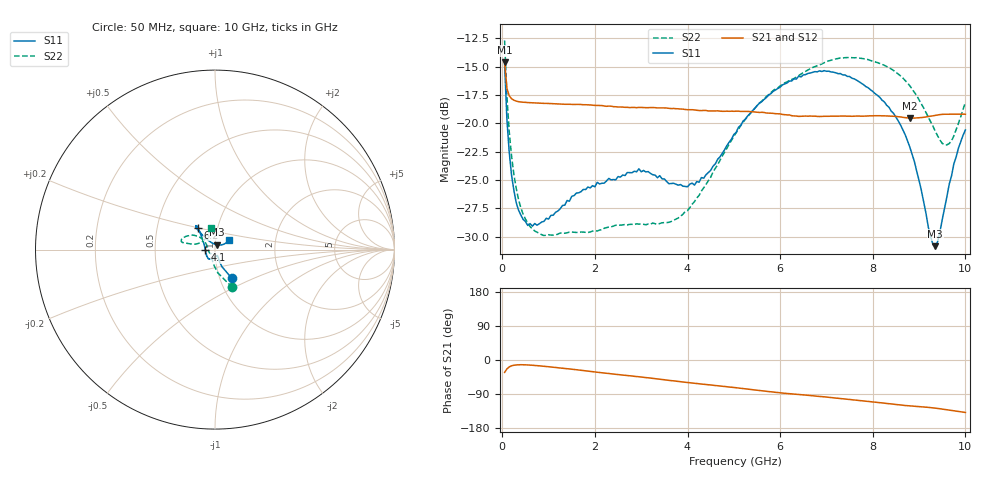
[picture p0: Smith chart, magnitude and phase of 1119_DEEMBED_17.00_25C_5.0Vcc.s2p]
!Hittite Microwave Corp.
!Digital Attenuator/PhaseShifter Rev 1.4.0
!Filename: C:\DATA\DATA\1119_DEEMBED_17.00_25C_5.0Vcc.s2p
!VNA ID: Agilent Technologies,N5224A,MY51441122,A.10.45.03
!Device type:
!2 Port Calibration.
!Temp(C): 25
!Lot Number:
!Serial Number:
!Operator:
!Misc:
!Attenuator:  17.000
# GHZ S DB R 50.0
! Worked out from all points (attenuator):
!   200 points, 50 MHz to 10 GHz, reference 50 ohm
!   highest |S21| = -14.61 dB at 50 MHz (marker M1); lowest = -19.5 dB at 8.8 GHz (marker M2)
!   lowest |S11| = -30.8 dB at 9.35 GHz (marker M3), VSWR 1.06, Z = 50.8 + j2.79 ohm
!   |S11| at or under -10 dB: start of sweep to end of sweep
!   |S22| runs from -29.9 to -12.7 dB; largest |S21 - S12| = 0.00046
!   S11 on the Smith chart (normalised r, x): 50 MHz: 1.14, -0.37; 4.1 GHz: 0.90, -0.00; 6.2 GHz: 0.81, +0.20; 10 GHz: 1.16, +0.12
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0.05  -14.75 -59.7  -14.61 -32.7  -14.61 -32.8  -12.68 -65.4
0.1  -19.67 -67.7  -16.91 -23.5  -16.91 -23.5  -17.62 -82.7
0.2  -24.57 -68.9  -17.82 -15.3  -17.82 -15.3  -22.90 -99.5
0.3  -26.98 -67.6  -18.03 -13.0  -18.02 -13.0  -25.71 -109.2
0.45  -28.47 -66.8  -18.13 -12.6  -18.13 -12.6  -28.01 -119.8
0.9  -28.64 -78.5  -18.23 -16.5  -18.25 -16.7  -29.89 -133.6
1.75  -25.82 -104.6  -18.35 -27.9  -18.35 -27.9  -29.59 -138.1
2.95  -24.00 -126.2  -18.59 -44.2  -18.60 -44.3  -28.89 -157.2
3.4  -24.61 -143.0  -18.63 -50.7  -18.63 -50.7  -28.83 -170.4
4.1  -25.27 -179.1  -18.79 -60.7  -18.80 -60.7  -27.13 161.4
4.5  -24.14 160.5  -18.90 -65.9  -18.92 -66.0  -24.75 147.4
5.05  -20.79 139.9  -18.92 -73.2  -18.94 -73.2  -20.82 140.5
5.55  -18.22 131.7  -19.03 -80.4  -19.04 -80.4  -18.21 142.6
6.2  -16.26 127.5  -19.25 -89.2  -19.27 -89.2  -16.20 148.4
6.7  -15.50 128.4  -19.36 -94.5  -19.37 -94.5  -15.07 154.9
7.5  -15.86 130.8  -19.36 -104.2  -19.37 -104.2  -14.19 163.9
8.35  -18.57 130.8  -19.35 -115.4  -19.35 -115.4  -15.08 167.5
8.8  -22.09 128.2  -19.53 -121.0  -19.52 -121.0  -16.68 167.2
9.25  -29.98 97.0  -19.36 -125.6  -19.38 -125.6  -19.86 160.9
9.35  -30.83 72.7  -19.29 -127.0  -19.31 -127.0  -20.69 155.8
9.65  -25.38 32.3  -19.19 -132.1  -19.20 -132.1  -21.78 126.5
10  -20.58 34.2  -19.19 -138.4  -19.20 -138.4  -18.12 99.5
